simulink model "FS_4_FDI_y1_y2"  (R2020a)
settings: Solver=VariableStepAuto  StartTime=0.0  StopTime=30  RelTol=1e-3
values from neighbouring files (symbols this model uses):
  C = 6.3000e-04    (= 0.00063)    [maglev_init.m]
  g = 9.80    (= 9.8)    [maglev_init.m]
  K = 1.0e+03 * [-2.4567   -0.1235    0.0237]    [maglev_init.m]
  L1 = 0.6000    (= 0.6)    [maglev_init.m]
  m = 0.0300    (= 0.03)    [maglev_init.m]
  mpert = 0    [maglev_init.m]
  R = 45    [maglev_init.m]
  Ts = 0.005    [maglev_init.m]    (also in train_net.m)
  x1_0 = 0.1    [maglev_init.m]
  x1_d = 0.05    [maglev_init.m]
  x2_0 = 0    [maglev_init.m]
  x2_d = 0    [maglev_init.m]
  x3_0 = 0.2    [maglev_init.m]
libraries: fuzblock x2

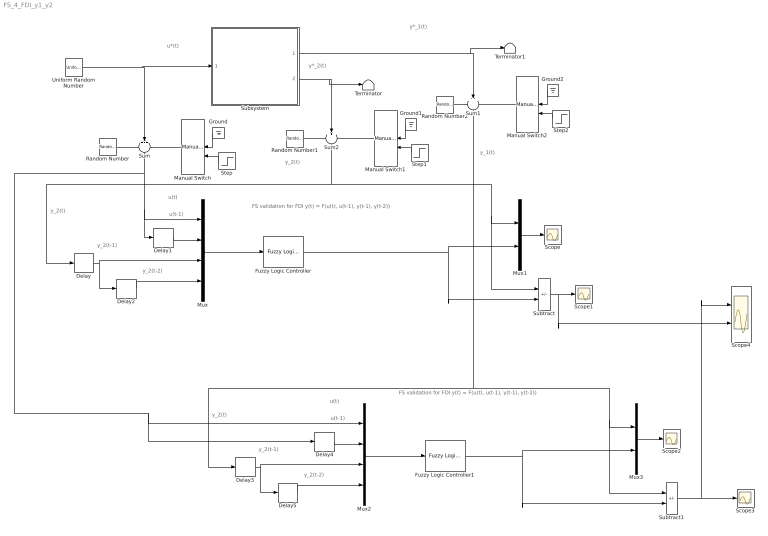
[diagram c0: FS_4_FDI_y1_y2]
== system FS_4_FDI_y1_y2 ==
  note: y_2(t)
  note: y_2(t-1)
  note: FS validation for FDI y(t) = F(u(t), u(t-1), y(t-1), y(t-2))
  note: y_2(t)
  note: y*_1(t)
  note: u(t)
  note: u*(t)
  note: y*_2(t)
  note: y_1(t)
  note: u(t-1)
  note: y_2(t-2)
  note: u(t)
  note: y_2(t)
  note: u(t-1)
  note: FS validation for FDI y(t) = F(u(t), u(t-1), y(t-1), y(t-2))
  note: y_2(t-2)
  note: y_2(t-1)
  Delay{,1..5} (6 alike) : Delay  DelayLength=1  SampleTime=Ts
  Fuzzy Logic Controller : fuzblock/Fuzzy Logic  Controller  FIS=FIS03  OutputSampleNumber=101  DataType=double  FuzzifiedInputs=off  RuleFiringStrengths=off  RuleOutputs=off  AggregatedOutputs=off  SimulateUsing=Interpreted execution  OutOfRangeInputValueMessage=warning  NoRuleFiredMessage=warning  EmptyOutputFuzzySetMessage=warning
  Fuzzy Logic Controller1 : fuzblock/Fuzzy Logic  Controller  FIS=FIS04  OutputSampleNumber=101  DataType=double  FuzzifiedInputs=off  RuleFiringStrengths=off  RuleOutputs=off  AggregatedOutputs=off  SimulateUsing=Interpreted execution  OutOfRangeInputValueMessage=warning  NoRuleFiredMessage=warning  EmptyOutputFuzzySetMessage=warning
  Ground : Ground
  Ground1 : Ground
  Ground2 : Ground
  Manual Switch : ManualSwitch
  Manual Switch1 : ManualSwitch
  Manual Switch2 : ManualSwitch
  Mux : Mux
  Mux1 : Mux  Inputs=2
  Mux2 : Mux
  Mux3 : Mux  Inputs=2
  Random Number : RandomNumber  Variance=1e-9  Seed=1  SampleTime=Ts
  Random Number1 : RandomNumber  Variance=1e-6  Seed=3  SampleTime=Ts
  Random Number2 : RandomNumber  Variance=1e-9  Seed=2  SampleTime=Ts
  Scope{,1..3} (4 alike) : Scope
  Scope4 : Scope  NumInputPorts=2
  Step : Step  Time=15  SampleTime=0
  Step1 : Step  Time=15  SampleTime=0
  Step2 : Step  Time=15  SampleTime=0
  Subsystem : Subsystem
  Subtract : Sum  Inputs=+-
  Subtract1 : Sum  Inputs=+-
  Sum : Sum  Inputs=+++
  Sum1 : Sum  Inputs=+++
  Sum2 : Sum  Inputs=+++
  Terminator : Terminator
  Terminator1 : Terminator
  Uniform Random Number : UniformRandomNumber  Minimum=x1_d*0.9  Maximum=x1_d*1.1  Seed=1  SampleTime=0.5
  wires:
  Uniform Random Number/1 -> Subsystem/1(In1), Sum/2
  Subsystem/1(Out1) -> Terminator1/1, Sum1/2
  Subsystem/2(Out2) -> Terminator/1, Sum2/2
  Random Number/1 -> Sum/1
  Manual Switch/1 -> Sum/3
  Manual Switch2/1 -> Sum1/3
  Manual Switch1/1 -> Sum2/3
  Random Number1/1 -> Sum2/1
  Ground/1 -> Manual Switch/1
  Step/1 -> Manual Switch/2
  Ground1/1 -> Manual Switch1/1
  Step1/1 -> Manual Switch1/2
  Random Number2/1 -> Sum1/1
  Ground2/1 -> Manual Switch2/1
  Step2/1 -> Manual Switch2/2
  Delay1/1 -> Mux/2
  Delay/1 -> Delay2/1, Mux/3
  Delay2/1 -> Mux/4
  Mux/1 -> Fuzzy Logic Controller/1
  Fuzzy Logic Controller/1 -> Subtract/2, Mux1/2
  Mux1/1 -> Scope/1
  Mux3/1 -> Scope2/1
  Mux2/1 -> Fuzzy Logic Controller1/1
  Fuzzy Logic Controller1/1 -> Mux3/2, Subtract1/2
  Delay5/1 -> Mux2/4
  Delay3/1 -> Delay5/1, Mux2/3
  Subtract1/1 -> Scope3/1, Scope4/1
  Sum2/1 -> Delay/1, Subtract/1, Mux1/1
  Delay4/1 -> Mux2/2
  Sum1/1 -> Mux3/1, Subtract1/1, Delay3/1
  Sum/1 -> Mux2/1, Delay4/1, Delay1/1, Mux/1
  Subtract/1 -> Scope4/2, Scope1/1

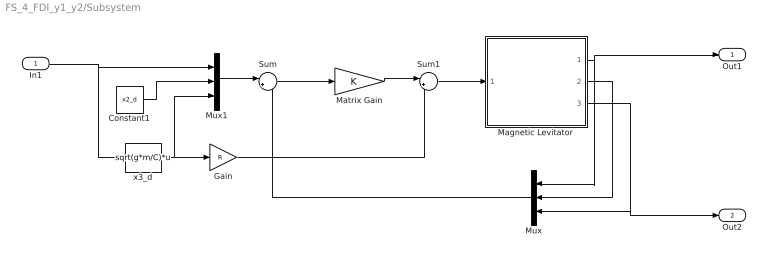
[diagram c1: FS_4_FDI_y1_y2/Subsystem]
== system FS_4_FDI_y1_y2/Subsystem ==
  In1 : Inport
  Constant1 : Constant  Value=x2_d
  Gain : Gain  Gain=R
  Magnetic Levitator : Subsystem  mask{m=m+mpert, R=R, L1=L1, C=C, g=g}
      mask prompts: m "ball's mass (m)"; R "Electromagnet's resistance (R)"; L1 "Electromagnet's inductance (L1)"; C "Magnetic force constant (C)"; g "Gravitational acceleration (g)"
  Matrix Gain : Gain  Gain=K  Multiplication=Matrix(K*u)  SaturateOnIntegerOverflow=on
  Mux : Mux  Inputs=3
  Mux1 : Mux  Inputs=3
  Sum : Sum  Inputs=|+-  InputSameDT=on  SaturateOnIntegerOverflow=on
  Sum1 : Sum  Inputs=|++  InputSameDT=on  SaturateOnIntegerOverflow=on
  x3_d : Fcn  Expr=sqrt(g*m/C)*u
  Out1 : Outport
  Out2 : Outport  Port=2
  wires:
  In1/1 -> x3_d/1, Mux1/1
  Magnetic Levitator/2(x2) -> Mux/2
  x3_d/1 -> Mux1/3, Gain/1
  Mux1/1 -> Sum/1
  Gain/1 -> Sum1/2
  Mux/1 -> Sum/2
  Constant1/1 -> Mux1/2
  Sum/1 -> Matrix Gain/1
  Sum1/1 -> Magnetic Levitator/1(u)
  Magnetic Levitator/1(x1) -> Out1/1, Mux/1
  Magnetic Levitator/3(x3) -> Out2/1, Mux/3
  Matrix Gain/1 -> Sum1/1

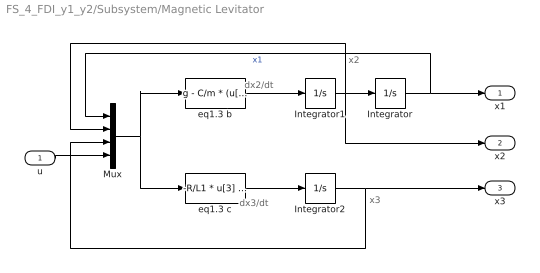
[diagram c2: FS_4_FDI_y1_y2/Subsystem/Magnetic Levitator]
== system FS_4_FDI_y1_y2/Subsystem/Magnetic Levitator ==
  note: x2
  note: x3
  note: dx2/dt
  note: dx3/dt
  u : Inport
  Integrator : Integrator  InitialCondition=x1_0
  Integrator1 : Integrator  InitialCondition=x2_0
  Integrator2 : Integrator  InitialCondition=x3_0
  Mux : Mux
  eq1.3 b : Fcn  Expr=g - C/m * (u[3] / u[1])^2
  eq1.3 c : Fcn  Expr=-R/L1 * u[3] + (2*C)/L1 * ( u[2] * u[3] / u[1]^2 ) + 1/L1 * u[4]
  x1 : Outport
  x2 : Outport  Port=2
  x3 : Outport  Port=3
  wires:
  eq1.3 b/1 -> Integrator1/1
  Integrator1/1 -> Integrator/1, Mux/2, x2/1
  eq1.3 c/1 -> Integrator2/1
  Mux/1 -> eq1.3 b/1, eq1.3 c/1
  Integrator/1 -> Mux/1, x1/1  "x1"
  Integrator2/1 -> Mux/3, x3/1
  u/1 -> Mux/4
